// TwinCAT 3 PLC project cutter
// libraries:
//   Tc2_Math, * (Beckhoff Automation GmbH)
//   Tc2_MC2, * (Beckhoff Automation GmbH)
//   Tc2_MC2_Camming, * (Beckhoff Automation GmbH)
//   Tc2_Standard, * (Beckhoff Automation GmbH)
//   Tc2_System, * (Beckhoff Automation GmbH)
//   Tc3_Module, * (Beckhoff Automation GmbH)
// project tree:
//   Data types/ step.TcDUT
//   Global Variables/ Global_Variables.TcGVL, TwinCAT_Configuration.TcGVL, Variable_Configuration.TcGVL
//   / PlcTask.TcTTO
//   POUs/ MAIN.TcPOU
// real-time tasks:
//   TASK PlcTask: cycle T#10ms, priority 21, ADS port 351
// motion (NC):
//   TASK NC-Task 1 SAF: cycle T#2ms, priority 4, ADS port 501
//   TASK NC-Task 1 SVB: cycle T#10ms, priority 8, ADS port 511
//   AXIS slave12 (id 1)
//     General: UnitFlags=#x00000004
//     Dynamic: AccelerationMaximum=0, DecelerationMaximum=0, Acceleration=13526.4, Deceleration=13526.4, Jerk=80097.2
//     Velo: RefSearch=44.7893333333333, RefSync=44.7893333333333, SlowManual=223.946666666667, FastManual=1343.68, Fast=4478.93333333333, Maximum=4478.93
//     encoder EncType=19
//       EncPara: ScaleFactorNumerator=239, ScaleFactorDenominator=1048576, Offset=7.889, ModuloFactor=239, Inverse=true, MaxCount=#xffffffff
//     drive DrvType=16
//       DrvPara: Inverse=true, MaxCount=#xffffffff, DriveControlDWord=#x00000100
//         Analog: VeloReferenz=4926.82666666667, VeloScale=32, SmoothingFilterOrder=0, SmoothingFilterTime=0
//         TimeComp: TaskDelayCycles=1
//     controller CtrType=1
//       CtrPara: PriorControlFactor=1
//         PosDiffControl: Range=20
//         Observer: BandWidth=20
//   AXIS master11 (id 2)
//     Dynamic: AccelerationMaximum=0, DecelerationMaximum=0, Acceleration=7371.52, Deceleration=7371.52, Jerk=22114.6
//     Velo: RefSearch=49.1434666666667, RefSync=49.1434666666667, SlowManual=245.717333333333, FastManual=1474.304, Fast=4914.34666666667, Maximum=4914.35
//     encoder EncType=19
//       EncPara: ScaleFactorNumerator=166.4, ScaleFactorDenominator=1048576, MaxCount=#xffffffff
//     drive DrvType=16
//       DrvPara: MaxCount=#xffffffff, DriveControlDWord=#x00000100
//         Analog: VeloReferenz=5405.78133333333, VeloScale=32, SmoothingFilterOrder=0, SmoothingFilterTime=0
//         TimeComp: TaskDelayCycles=1
//     controller CtrType=1
//       CtrPara: PriorControlFactor=1
//         PosDiffControl: Range=10
//         Observer: BandWidth=20
// I/O:
//   DEVICE Device 1 (EtherCAT), AmsNetId 169.254.146.161.2.1
//     Term 1 (EK1200) [EK1200-5000 EtherCAT Power supply (2A E-Bus)]
//       Term 2 (EL1004) [EL1004 4Ch. Dig. Input 24V, 3ms]
//       Term 3 (EL2024) [EL2024 4Ch. Dig. Output 24V, 2A]
//       Term 4 (EL1004) [EL1004 4Ch. Dig. Input 24V, 3ms]
//       Term 5 (EL2004) [EL2004 4Ch. Dig. Output 24V, 0.5A]
//       Term 6 (EL1259) [EL1259 8Ch. Dig Input 24V/8Ch. Dig. Output 24V with Multi-Time-Stamp]
//       Term 7 (EL6900) [EL6900, TwinSAFE PLC]
//       Term 8 (EL1904) [EL1904, 4 Ch. Safety Input 24V, TwinSAFE]
//         modules: Module 1 (FSOES)
//       Term 9 (EL2904) [EL2904, 4 Ch. Safety Output 24V, 0.5A, TwinSAFE]
//         modules: Module 1 (FSOES), Module 2 (DO)
//       Term 10 (EL3255) [EL3255 5Ch. potentiometer measurement with sensor supply]
//       Term 11 (EL7201-9014) [EL7201-9014 1Ch. MDP742 Servo motor output stage with OCT (50V, 4A)  and STO input]
//       Term 12 (EL7201-9014) [EL7201-9014 1Ch. MDP742 Servo motor output stage with OCT (50V, 4A)  and STO input]
//       Term 13 (EL6731-0010) [EL6731-0010 PROFIBUS DP Slave]
//       Term 14 (EL9011) [EL9011 End Terminal]
//   DEVICE Device 4 (COM Port)
// variable links:
//   NC-Task 1 SAF/Axes/master11 <-> Device 1 (EtherCAT)/Term 1 (EK1200)/Term 11 (EL7201-9014)
//     master11_Drive/Inputs/master11_Drive_In/nDataIn1 <-> DRV Following error actual value/Following error actual value
//     master11_Drive/Inputs/master11_Drive_In/nDcOutputTime <-> InfoData/DcOutputShift
//     master11_Drive/Inputs/master11_Drive_In/nState1 <-> DRV Statusword/Statusword
//     master11_Drive/Inputs/master11_Drive_In/nState2 <-> DRV Statusword/Statusword @bit 8
//     master11_Drive/Inputs/master11_Drive_In/nState4 @bit 1 <-> WcState/InputToggle
//     master11_Drive/Inputs/master11_Drive_In/nState4 <-> WcState/WcState
//     master11_Drive/Outputs/master11_Drive_Out/nCtrl1 <-> DRV Controlword/Controlword
//     master11_Drive/Outputs/master11_Drive_Out/nCtrl2 <-> DRV Controlword/Controlword @bit 8
//     master11_Drive/Outputs/master11_Drive_Out/nDataOut1 <-> DRV Target position/Target position
//     master11_Enc/Inputs/master11_Enc_In/nDataIn1 <-> FB Position/Position
//     master11_Enc/Inputs/master11_Enc_In/nDcInputTime <-> InfoData/DcInputShift
//     master11_Enc/Inputs/master11_Enc_In/nState4 @bit 1 <-> WcState/InputToggle
//     master11_Enc/Inputs/master11_Enc_In/nState4 <-> WcState/WcState
//   NC-Task 1 SAF/Axes/slave12 <-> Device 1 (EtherCAT)/Term 1 (EK1200)/Term 12 (EL7201-9014)
//     slave12_Drive/Inputs/slave12_Drive_In/nDataIn1 <-> DRV Following error actual value/Following error actual value
//     slave12_Drive/Inputs/slave12_Drive_In/nDcOutputTime <-> InfoData/DcOutputShift
//     slave12_Drive/Inputs/slave12_Drive_In/nState1 <-> DRV Statusword/Statusword
//     slave12_Drive/Inputs/slave12_Drive_In/nState2 <-> DRV Statusword/Statusword @bit 8
//     slave12_Drive/Inputs/slave12_Drive_In/nState4 @bit 1 <-> WcState/InputToggle
//     slave12_Drive/Inputs/slave12_Drive_In/nState4 <-> WcState/WcState
//     slave12_Drive/Outputs/slave12_Drive_Out/nCtrl1 <-> DRV Controlword/Controlword
//     slave12_Drive/Outputs/slave12_Drive_Out/nCtrl2 <-> DRV Controlword/Controlword @bit 8
//     slave12_Drive/Outputs/slave12_Drive_Out/nDataOut1 <-> DRV Target position/Target position
//     slave12_Enc/Inputs/slave12_Enc_In/nDataIn1 <-> FB Position/Position
//     slave12_Enc/Inputs/slave12_Enc_In/nDcInputTime <-> InfoData/DcInputShift
//     slave12_Enc/Inputs/slave12_Enc_In/nState4 @bit 1 <-> WcState/InputToggle
//     slave12_Enc/Inputs/slave12_Enc_In/nState4 <-> WcState/WcState
//   cutter/cutter Instance <-> Device 1 (EtherCAT)/Term 1 (EK1200)/Term 6 (EL1259)
//     PlcTask Inputs/MAIN.bEL1259_input <-> TSI Inputs Channel 1/Input
//   cutter/cutter Instance <-> NC-Task 1 SAF/Axes/master11
//     PlcTask Inputs/MAIN.master.NcToPlc <-> Outputs/master11_ToPlc
//     PlcTask Outputs/MAIN.master.PlcToNc <-> Inputs/master11_FromPlc
//   cutter/cutter Instance <-> NC-Task 1 SAF/Axes/slave12
//     PlcTask Inputs/MAIN.slave.NcToPlc <-> Outputs/slave12_ToPlc
//     PlcTask Outputs/MAIN.slave.PlcToNc <-> Inputs/slave12_FromPlc

CONFIGURATION cutter
    RESOURCE PLC ON TwinCAT3
        TASK PlcTask(INTERVAL := T#10ms, PRIORITY := 21);
        PROGRAM MAIN WITH PlcTask : MAIN;
    END_RESOURCE
END_CONFIGURATION

// ---- Data types/step.TcDUT
TYPE step :
(
	init,
	homing:=100,
	creating_cam:=200,
	camming:=300,
	insync:=400,
	error:=500,
	reset:=600
);
END_TYPE

// ---- Global Variables/Global_Variables.TcGVL
{attribute 'Tc2GvlVarNames'}
VAR_GLOBAL
END_VAR

// ---- Global Variables/TwinCAT_Configuration.TcGVL
{attribute 'Tc2GvlVarNames'}
(* Generated automatically by TwinCAT - (read only) *)
VAR_CONFIG
	MAIN.master.PlcToNc AT %QB0 : PLCTONC_AXIS_REF;
	MAIN.master.NcToPlc AT %IB1 : NCTOPLC_AXIS_REF;
	MAIN.slave.PlcToNc AT %QB128 : PLCTONC_AXIS_REF;
	MAIN.slave.NcToPlc AT %IB129 : NCTOPLC_AXIS_REF;
	MAIN.bEL1259_input AT %IX0.0 : BOOL;
END_VAR

// ---- Global Variables/Variable_Configuration.TcGVL
{attribute 'Tc2GvlVarNames'}
VAR_CONFIG
END_VAR

// ---- POUs/MAIN.TcPOU
PROGRAM MAIN
VAR
	master,slave:				axis_ref;
	power_m,power_s:		MC_Power;
	process:					step;
	move_m:				MC_MoveVelocity;
	move_s:					MC_MoveModulo;
	stop_m:					MC_Stop;
	setpos_m:				MC_SetPosition;
	reset_s,reset_m:			MC_Reset;

	bEL1259_input AT%I*:	BOOL;

	camin:					MC_CamIn;
	camout:					MC_CamOut;
	camtableselect:			MC_CamTableSelect;
	cam_table1:				MC_CAM_REF;
	table1:					ARRAY[1..4]OF MC_MotionFunctionPoint;

END_VAR

axis_basic();
cam();
master();
slave();
CASE process OF
init:
	reset_m.Execute:=FALSE;
	reset_s.Execute:=FALSE;
	camin.Execute:=FALSE;
	move_m.Execute:=FALSE;
	move_s.Execute:=FALSE;
	camout.Execute:=FALSE;
	IF power_m.status AND power_s.status THEN
		process:=homing;
	END_IF
	IF slave.Status.Error OR master.Status.Error THEN
		process:=error;
	END_IF

homing:
	move_m.Execute:=TRUE;
	move_s.Execute:=TRUE;
	IF move_m.InVelocity AND	bEL1259_input  THEN
		stop_m.Execute:=TRUE;
	END_IF
	IF stop_m.Done AND move_s.Done THEN
		setpos_m.Execute:=TRUE;
		move_m.Execute:=FALSE;
		move_s.Execute:=FALSE;
		stop_m.Execute:=FALSE;
		IF	setpos_m.Done THEN
			setpos_m.Execute:=FALSE;
			process:=creating_cam;
		END_IF
	END_IF
	IF slave.Status.Error OR master.Status.Error THEN
		process:=error;
	END_IF

creating_cam:
	camtableselect.Execute:=TRUE;
	IF camtableselect.Done THEN
		camtableselect.Execute:=FALSE;
		move_m.Execute:=TRUE;
		IF master.Status.Moving THEN
			process:=camming;
			move_m.Execute:=FALSE;
		END_IF
	END_IF
	IF slave.Status.Error OR master.Status.Error THEN
		process:=error;
	END_IF

camming:
	camout.Execute:=false;
	camin.Execute:=bEL1259_input ;

	IF camin.InSync THEN
		process:=InSync;
	END_IF
	IF slave.Status.Error OR master.Status.Error THEN
		process:=error;
	END_IF

InSync:
	(*IF   slave.NcToPlc.ActPos <0.1 OR slave.NcToPlc.ActPos>16.63 THEN*)
	IF NOT slave.Status.Moving THEN
		camout.Execute:=TRUE;
		IF camout.Done THEN
			process:=camming;
		END_IF
	END_IF
	IF slave.Status.Error OR master.Status.Error THEN
		process:=error;
	END_IF

error:
	camout.Execute:=slave.Status.Coupled;
	IF NOT slave.Status.Coupled THEN
		IF master.Status.Error OR slave.Status.Error THEN
			process:=reset;
		ELSE
			process:=init;
		END_IF
	END_IF

reset:
	reset_m.Execute:=TRUE;
	reset_s.Execute:=TRUE;
	camin.Execute:=FALSE;
	move_m.Execute:=FALSE;
	move_s.Execute:=FALSE;
	IF reset_m.Done AND reset_s.Done THEN
		process:=init;
	ELSIF reset_m.Error OR reset_s.Error THEN
		process:=init;
	END_IF





END_CASE

ACTION axis_basic:
power_m(
	Enable:=TRUE ,
	Enable_Positive:= TRUE,
	Enable_Negative:=TRUE ,
	Axis:=master , );
power_S(
	Enable:=TRUE ,
	Enable_Positive:= TRUE,
	Enable_Negative:=TRUE ,
	Axis:=slave , );
move_m(
	Execute:=move_m.Execute ,
	Velocity:=300 ,
	Direction:=1 ,
	Axis:=master , );
move_s(
	Execute:=move_s.Execute ,
	Position:=239 ,
	Velocity:=300,
	Axis:=slave , );
setpos_m(
	Execute:= setpos_m.Execute,
	Position:= 0,
	Axis:= master, );
stop_m(
	Execute:=stop_m.Execute ,
	Axis:=master ,);
reset_m(
	Execute:=reset_m.Execute ,
	Axis:=master , );
reset_s(
	Execute:=reset_s.Execute ,
	Axis:=slave , );
END_ACTION

ACTION cam:
camin(
	Execute:=camin.Execute ,
	StartMode:= MC_STARTMODE_relative,
	CamTableID:=1 ,
	Master:= master,
	Slave:=slave , );
camout(
	Execute:=camout.Execute ,
	Slave:=slave , );
camtableselect(
	Execute:=camtableselect.Execute ,
	Periodic:=FALSE ,
	MasterAbsolute:= ,
	SlaveAbsolute:= ,
	CamTableID:= 1,
	Master:=master ,
	Slave:=slave ,
	CamTable:= cam_table1, );

cam_table1.ArraySize:=SIZEOF(table1);
cam_table1.NoOfColumns:=1;
cam_table1.NoOfRows:=4;
cam_table1.pArray:=ADR(table1);
cam_table1.TableType:=22;(*MC_TableType_TABULARTYPE_MOTIONFUNC*)

table1[1].FunctionType:=MOTIONFUNCTYPE_POLYNOM1;
table1[1].MasterPos:=0;
table1[1].SlavePos:=0;
table1[1].PointIndex:=1;
table1[1].PointType:=MOTIONPOINTTYPE_REST;

table1[2].FunctionType:=MOTIONFUNCTYPE_POLYNOM1;
table1[2].MasterPos:=170.3;
table1[2].SlavePos:=55.75;
table1[2].PointIndex:=2;
table1[2].PointType:=MOTIONPOINTTYPE_VELOCITY;
table1[2].SlaveVelo:=300;

table1[3].FunctionType:=MOTIONFUNCTYPE_POLYNOM5;
table1[3].MasterPos:=179.3;
table1[3].SlavePos:=60.75;
table1[3].PointIndex:=3;
table1[3].PointType:=MOTIONPOINTTYPE_VELOCITY;
table1[3].SlaveVelo:=300;

table1[4].FunctionType:=MOTIONFUNCTYPE_POLYNOM3;
table1[4].MasterPos:=357.55;
table1[4].SlavePos:=239;
table1[4].PointIndex:=4;
table1[4].PointType:=MOTIONPOINTTYPE_REST;
END_ACTION

END_PROGRAM
